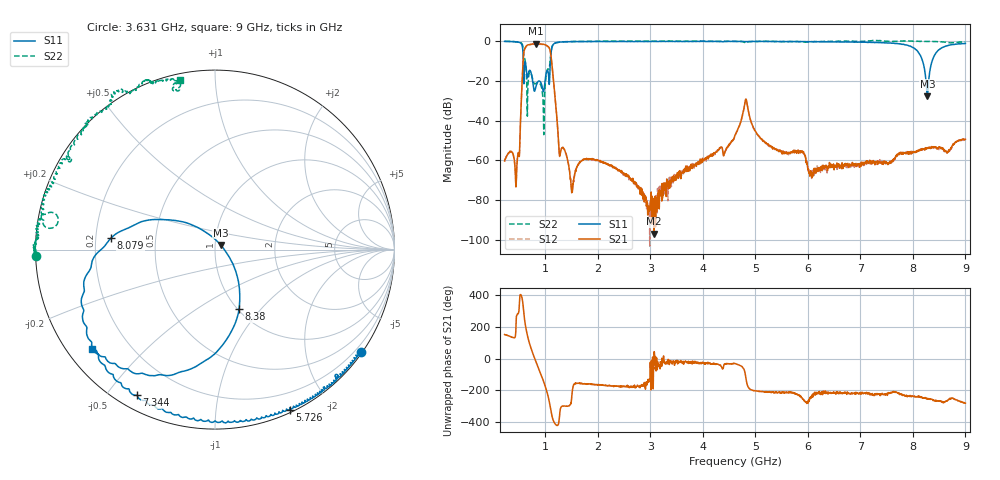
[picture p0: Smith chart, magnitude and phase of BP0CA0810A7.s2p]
!Agilent Technologies,E8358A,US41080443,A.07.50.56
!Agilent E8358A: A.07.50.56
!Date: Thursday, November 09, 2017 08:50:35
!Correction: S11(Full 2 Port(1,2))
!S21(Full 2 Port(1,2))
!S12(Full 2 Port(1,2))
!S22(Full 2 Port(1,2))
!S2P File: Measurements: S11, S21, S12, S22:
# Hz S  dB  R 50
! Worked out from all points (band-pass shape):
!   1601 points, 225 MHz to 9 GHz, reference 50 ohm
!   highest |S21| = -1.28 dB at 817.3 MHz (marker M1); lowest = -97.0 dB at 3.071 GHz (marker M2)
!   |S21| within 3 dB of the highest: 601.4 MHz to 1.088 GHz (486.6 MHz wide, 57.6 % of centre)
!   lowest |S11| = -27.8 dB at 8.276 GHz (marker M3), VSWR 1.09, Z = 53.3 + j2.68 ohm
!   |S11| at or under -10 dB: 581.8 MHz to 1.097 GHz (515.6 MHz wide, 61.4 % of centre); 8.185 GHz to 8.366 GHz (181.1 MHz wide, 2.19 % of centre)
!   |S22| runs from -47.1 to 0.4 dB; largest |S21 - S12| = 0.016
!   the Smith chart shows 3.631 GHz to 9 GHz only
!   S11 on the Smith chart (normalised r, x): 3.631 GHz: 0.04, -3.17; 5.726 GHz: 0.03, -1.57; 7.344 GHz: 0.06, -0.60; 8.079 GHz: 0.26, +0.05; 8.38 GHz: 1.01, -0.77; 9 GHz: 0.07, -0.35
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2.25e8  -0.08 -20.6  -60.34 151.2  -60.36 153.0  -0.04 153.6
4.663125e8  -0.35 -62.5  -59.72 -80.6  -59.91 -82.9  -0.33 105.5
6.089062e8  -10.57 -90.7  -3.75 -123.7  -3.91 -123.4  -8.96 21.5
7.07625e8  -14.70 -91.7  -1.63 86.0  -1.79 86.1  -15.51 85.9
8.173125e8  -23.32 87.7  -1.28 -16.4  -1.43 -16.2  -21.28 60.0
9.928125e8  -20.68 114.0  -1.75 -168.9  -1.90 -168.8  -24.10 36.9
1.288969e9  -0.42 60.8  -55.92 44.6  -56.20 44.4  -0.41 -103.1
1.513828e9  -0.24 33.4  -76.10 152.7  -75.02 149.5  -0.10 -136.7
1.689328e9  -0.19 21.4  -60.30 -157.1  -60.45 -156.5  -0.07 -150.3
3.071391e9  -0.18 -24.2  -96.98 43.3  -87.34 -49.4  0.02 -173.9
3.153656e9  -0.14 -25.6  -80.26 -36.5  -77.21 -1.1  0.06 -174.9
3.630797e9  -0.07 -35.0  -66.48 -35.1  -66.89 -24.4  -0.02 -178.1
4.6125e9  -0.06 -49.1  -47.43 -32.0  -47.71 -30.8  -0.01 171.6
4.820906e9  -0.19 -51.9  -29.14 -124.4  -29.37 -124.0  -1.04 169.7
5.725828e9  -0.15 -65.0  -55.14 142.9  -55.15 144.0  -0.09 151.0
6.076828e9  -0.23 -72.7  -68.74 129.7  -67.90 126.8  -0.28 147.1
7.343719e9  -0.71 -118.3  -60.45 136.2  -61.06 131.9  0.27 121.4
7.541156e9  -0.90 -129.8  -61.21 145.0  -61.10 141.6  -0.08 118.6
8.078625e9  -4.67 173.8  -55.19 119.7  -55.42 122.8  -0.02 111.1
8.276062e9  -27.77 37.9  -53.72 104.3  -53.62 107.5  -0.12 108.7
8.380266e9  -8.92 -68.1  -53.57 99.8  -53.34 98.5  -0.16 105.9
9e9  -1.10 -141.1  -49.41 78.7  -49.41 78.6  -0.30 101.7
